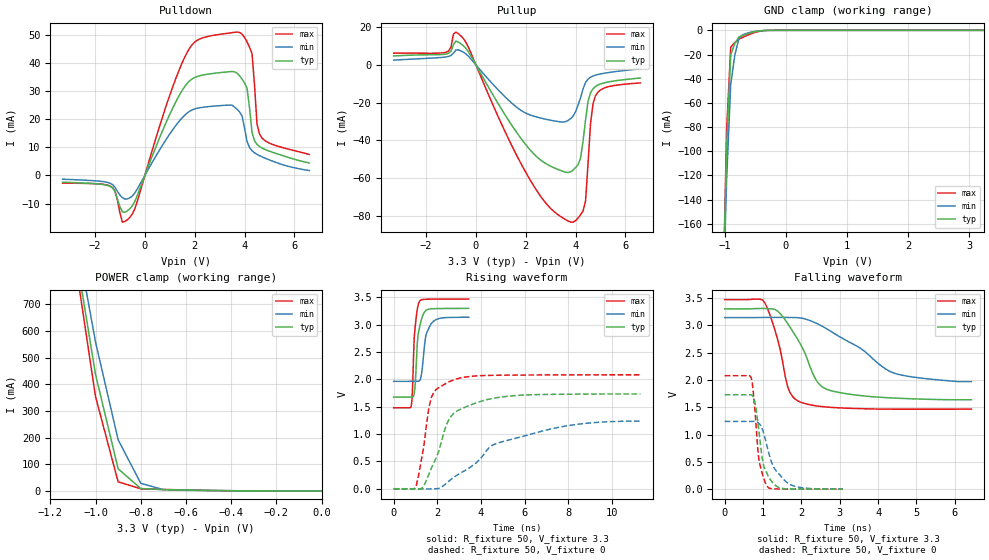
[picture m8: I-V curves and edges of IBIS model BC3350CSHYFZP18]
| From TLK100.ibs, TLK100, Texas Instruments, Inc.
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|   Model Cell BC3350CSHYFZP18
[Model]   BC3350CSHYFZP18
Model_type   I/O
Polarity   Non-Inverting
Enable   Active-Low
Vinl =  0.8V
Vinh =  2V
Cref =  15.0000pF
Rref =  100.0000M
Vref =  0V
Vmeas =  1.65
C_comp   1.740586p   1.69194p   1.781861p
[Model Spec]
Vinl   0.8V   0.8V   0.8V
Vinh   2V   2V   2V
[Temperature Range]   25   125   -40
[Voltage Range]   3.3   3.14   3.47
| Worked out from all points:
|   slope of the pulldown table from 0 to 0.495 V, typ, clamps not added: 44 ohm
|   slope of the pullup table from 0 to 0.495 V, typ, clamps not added: 42.8 ohm
|   GND clamp passes 1 mA (typ) near -0.50 V on its own axis
|   POWER clamp passes 1 mA (typ) near -0.41 V on its own axis
|   rising waveform, R_fixture 50, V_fixture 3.3: 20-80 % time 200ps typ, 266ps min, 147ps max; typ from 1.68 V to 3.3 V
|   rising waveform, R_fixture 50, V_fixture 0: 20-80 % time 1.08ns typ, 3.31ns min, 507ps max; typ from 0 V to 1.73 V
|   falling waveform, R_fixture 50, V_fixture 3.3: 20-80 % time 710ps typ, 1.46ns min, 410ps max; typ from 3.3 V to 1.64 V
|   falling waveform, R_fixture 50, V_fixture 0: 20-80 % time 228ps typ, 423ps min, 170ps max; typ from 1.73 V to 0.001 V
[POWER_clamp]
|   voltage   I(typ)   I(min)   I(max)
-3.3V     15.06A     13.65A     16.18A
-1.067V   785.7mA    871.3mA    732.7mA
-1.033V   611.6mA    715.1mA    543.4mA
-1V       437.5mA    559mA      354.1mA
-900mV    83.07mA    192.2mA    34.28mA
-800mV    9.031mA    28.68mA    7.997mA
-700mV    4.77mA     4.795mA    5.583mA
-400mV    849.2uA    521.7uA    759.4uA
-11.55fV  112.9nA    207.8nA    237.1nA
[Pulldown]
|   voltage   I(typ)   I(min)   I(max)
-3.3V     -2.42mA    -1.355mA   -2.741mA
-1.4V     -3.865mA   -2.765mA   -3.734mA
-900mV    -12.98mA   -7.875mA   -16.62mA
-700mV    -12.57mA   -8.349mA   -15.75mA
1.7V      32.7mA     22.18mA    43.75mA
3.6V      36.79mA    24.25mA    50.83mA
3.9V      34.2mA     21.09mA    50.21mA
4.1V      30.98mA    12.06mA    47.43mA
4.3V      15.29mA    8.759mA    43.35mA
4.5V      11.02mA    7.483mA    18.29mA
4.6V      10.26mA    7.017mA    14.72mA
6.6V      4.411mA    1.71mA     7.433mA
[Pullup]
|   voltage   I(typ)   I(min)   I(max)
-3.3V     4.71mA     2.515mA    6.161mA
-1.2V     5.694mA    4.172mA    6.671mA
-1V       7.233mA    4.974mA    9.382mA
-900mV    10.66mA    6.234mA    16.33mA
-600mV    11.14mA    7.391mA    15.31mA
2.2V      -45.34mA   -26.6mA    -61.37mA
3.8V      -56.58mA   -28.42mA   -83.16mA
4.2V      -49.32mA   -17.48mA   -79.26mA
4.4V      -29.21mA   -9.305mA   -72.08mA
4.6V      -14.75mA   -6.54mA    -31.02mA
4.8V      -11.42mA   -5.442mA   -16.39mA
6.6V      -6.966mA   -2.122mA   -9.567mA
[GND_clamp]
|   voltage   I(typ)   I(min)   I(max)
-3.3V     -17.31A    -15.65A    -18.51A
-1.033V   -232.2mA   -237.1mA   -236.8mA
-966.7mV  -97.17mA   -123.2mA   -82.52mA
-900mV    -20.18mA   -44.67mA   -13.85mA
-833.3mV  -10.95mA   -20.55mA   -10.07mA
-766.7mV  -5.568mA   -6.818mA   -7.354mA
-700mV    -4.032mA   -3.482mA   -5.702mA
-500mV    -1.032mA   -814.8uA   -1.633mA
-300mV    -34.64uA   -47.12uA   -53.39uA
3.233V    81.09nA    2.44uA     207.5nA
[Ramp]
| variable   typ   min   max
dV/dt_f   1.004139/0.7133565n  0.7653473/1.650381n   1.209809/0.4114241n
dV/dt_r   1.04782/1.097234n   0.7654746/3.533183n   1.255633/0.5093347n
R_load = 50
[Rising Waveform]
R_fixture = 50
V_fixture = 3.3
V_fixture_min = 3.14
V_fixture_max = 3.47
|   time   V(typ)   V(min)   V(max)
0s        1.676V     1.965V     1.481V
804ps     1.677V     1.966V     1.508V
872ps     1.677V     1.966V     1.901V
944ps     1.741V     1.966V     2.778V
1.084ns   2.664V     1.965V     3.285V
1.188ns   2.951V     1.979V     3.43V
1.296ns   3.128V     2.154V     3.459V
1.472ns   3.259V     2.795V     3.466V
1.752ns   3.292V     3.035V     3.468V
3.44ns    3.299V     3.137V     3.47V
[Rising Waveform]
R_fixture = 50
V_fixture = 0
V_fixture_min = 0
V_fixture_max = 0
|   time   V(typ)   V(min)   V(max)
0s        49.57uV    25.45uV    83.1uV
1.036ns   -4.222mV   29.69uV    52.77mV
1.38ns    50.96mV    -2.554mV   769.9mV
1.612ns   263.9mV    -4.139mV   1.478V
1.728ns   377.7mV    -2.173mV   1.669V
2.532ns   1.266V     138.8mV    1.954V
3.224ns   1.483V     322.9mV    2.039V
4.84ns    1.673V     844.8mV    2.077V
8.072ns   1.729V     1.16V      2.083V
11.3ns    1.734V     1.238V     2.084V
[Falling Waveform]
R_fixture = 50
V_fixture = 3.3
V_fixture_min = 3.14
V_fixture_max = 3.47
|   time   V(typ)   V(min)   V(max)
0s        3.3V       3.14V      3.47V
1.048ns   3.308V     3.143V     3.408V
1.376ns   3.262V     3.144V     2.753V
1.64ns    3.035V     3.144V     1.88V
1.772ns   2.89V      3.142V     1.694V
1.968ns   2.663V     3.136V     1.596V
2.364ns   2.02V      3.045V     1.528V
2.692ns   1.82V      2.921V     1.502V
4.404ns   1.669V     2.127V     1.464V
6.432ns   1.636V     1.968V     1.464V
[Falling Waveform]
R_fixture = 50
V_fixture = 0
V_fixture_min = 0
V_fixture_max = 0
|   time   V(typ)   V(min)   V(max)
0s        1.728V     1.241V     2.077V
688ps     1.727V     1.241V     2.046V
780ps     1.623V     1.241V     1.51V
876ps     1.16V      1.215V     625.8mV
908ps     962.7mV    1.194V     474mV
1ns       479.3mV    1.063V     238.4mV
1.128ns   249.7mV    718.4mV    35.12mV
1.316ns   75.43mV    359.3mV    4.601mV
1.692ns   5.087mV    91.24mV    1.507mV
3.076ns   1.176mV    3.176mV    175.7uV
